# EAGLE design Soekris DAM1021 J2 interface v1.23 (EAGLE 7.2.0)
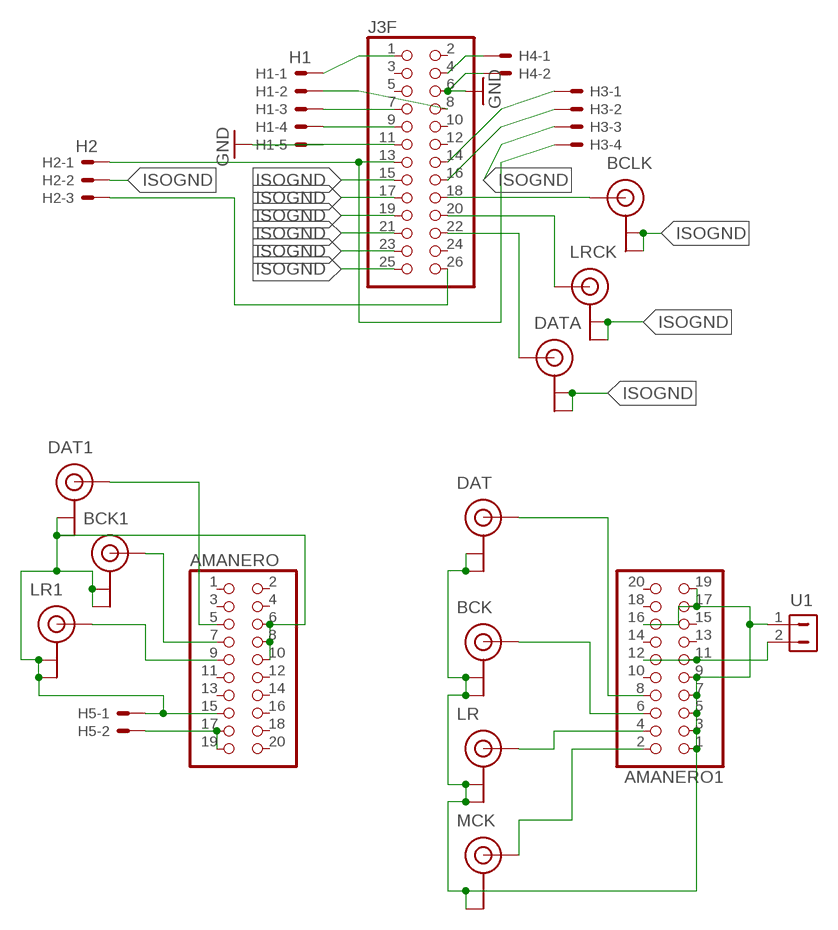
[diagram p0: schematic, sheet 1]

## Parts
AMANERO  PINHD-2X10_2.54  [2X10]
AMANERO1  PINHD-2X10_2.54  [2X10]
BCK  U.FL  [U.FL]
BCK1  U.FL  [U.FL]
BCLK  U.FL  [U.FL]
DAT  U.FL  [U.FL]
DAT1  U.FL  [U.FL]
DATA  U.FL  [U.FL]
H1  H1  22-23-2051  [22-23-2051]
H2  H2  22-23-2031  [22-23-2031]
H3  22-23-2041  [22-23-2041]
H4  22-23-2021  [22-23-2021]
H5  22-23-2021  [22-23-2021]
J3F  PINHD-2X13_2.54  [2X13]
LR  U.FL  [U.FL]
LR1  U.FL  [U.FL]
LRCK  U.FL  [U.FL]
MCK  U.FL  [U.FL]
U1  CON-2  [CON-2]

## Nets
GND: H1.5 H4.2 J3F.6 J3F.11
GNDA: AMANERO.6 AMANERO.8 AMANERO.10 AMANERO.15 BCK1.P$1(GND) BCK1.P$2(GND) DAT1.P$1(GND) DAT1.P$2(GND) H5.1 LR1.P$1(GND) LR1.P$2(GND)
H2: H2.3 J3F.26
ISOGND: BCLK.P$1(GND) BCLK.P$2(GND) DATA.P$1(GND) DATA.P$2(GND) H2.2 H3.3 J3F.15 J3F.17 J3F.19 J3F.21 J3F.23 J3F.25 LRCK.P$1(GND) LRCK.P$2(GND)
N$1: H2.1 H3.4 J3F.13
N$2: AMANERO1.2 MCK.P$3(SIGNAL)
N$3: H3.1 J3F.14
N$4: H3.2 J3F.16
N$5: BCLK.P$3(SIGNAL) J3F.18
N$6: H1.1 J3F.1
N$7: DATA.P$3(SIGNAL) J3F.22
N$8: AMANERO1.4 LR.P$3(SIGNAL)
N$9: J3F.20 LRCK.P$3(SIGNAL)
N$10: AMANERO1.8 DAT.P$3(SIGNAL)
N$11: H1.3 J3F.7
N$12: H1.2 J3F.8
N$13: H1.4 J3F.9
N$14: H4.1 J3F.4
N$15: AMANERO.17 AMANERO.19 H5.2
N$16: AMANERO1.6 BCK.P$3(SIGNAL)
N$17: AMANERO1.1 AMANERO1.3 AMANERO1.5 AMANERO1.7 AMANERO1.9 AMANERO1.16 AMANERO1.17 AMANERO1.19 BCK.P$1(GND) BCK.P$2(GND) DAT.P$1(GND) DAT.P$2(GND) LR.P$1(GND) LR.P$2(GND) MCK.P$1(GND) MCK.P$2(GND) U1.1
N$19: AMANERO.5 DAT1.P$3(SIGNAL)
N$20: AMANERO.7 BCK1.P$3(SIGNAL)
N$21: AMANERO.9 LR1.P$3(SIGNAL)
N$24: AMANERO1.11 AMANERO1.12 U1.2
Unconnected: AMANERO1.10 AMANERO1.13 AMANERO1.14 AMANERO1.15 AMANERO1.18 AMANERO1.20 AMANERO.1 AMANERO.2 AMANERO.3 AMANERO.4 AMANERO.11 AMANERO.12 AMANERO.13 AMANERO.14 AMANERO.16 AMANERO.18 AMANERO.20 J3F.2 J3F.3 J3F.5 J3F.10 J3F.12 J3F.24

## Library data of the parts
AMANERO AMANERO1 = pinhead-1:PINHD-2X10: PIN HEADER
BCK BCK1 BCLK DAT DAT1 DATA LR LR1 LRCK MCK = Dimdim:U.FL
H1 = con-molex:22-23-2051: .100" (2.54mm) Center Header - 5 Pin; MF: MOLEX; MPN: 22-23-2051; OC_FARNELL: 1462952; OC_NEWARK: 38C9178
H2 = con-molex:22-23-2031: .100" (2.54mm) Center Header - 3 Pin; MF: MOLEX; MPN: 22-23-2031; OC_FARNELL: 1462950; OC_NEWARK: 30C0862
H3 = con-molex:22-23-2041: .100" (2.54mm) Center Header - 4 Pin; MF: MOLEX; MPN: 22-23-2041; OC_FARNELL: 1462920; OC_NEWARK: 38C0355
H4 H5 = con-molex:22-23-2021: .100" (2.54mm) Center Header - 2 Pin; MF: MOLEX; MPN: 22-23-2021; OC_FARNELL: 1462926; OC_NEWARK: 25C3832
J3F = pinhead-1:PINHD-2X13: PIN HEADER
U1 = Dimdim:CON-2

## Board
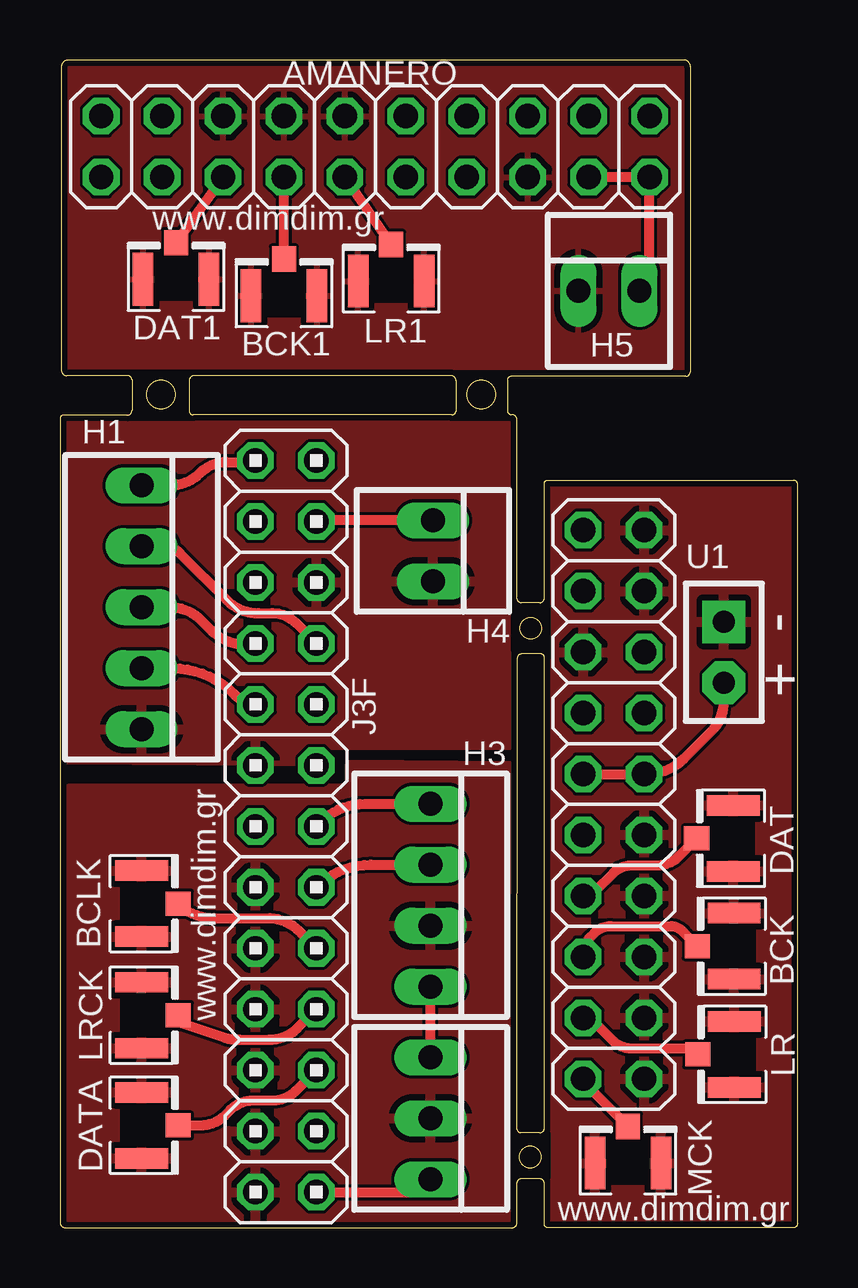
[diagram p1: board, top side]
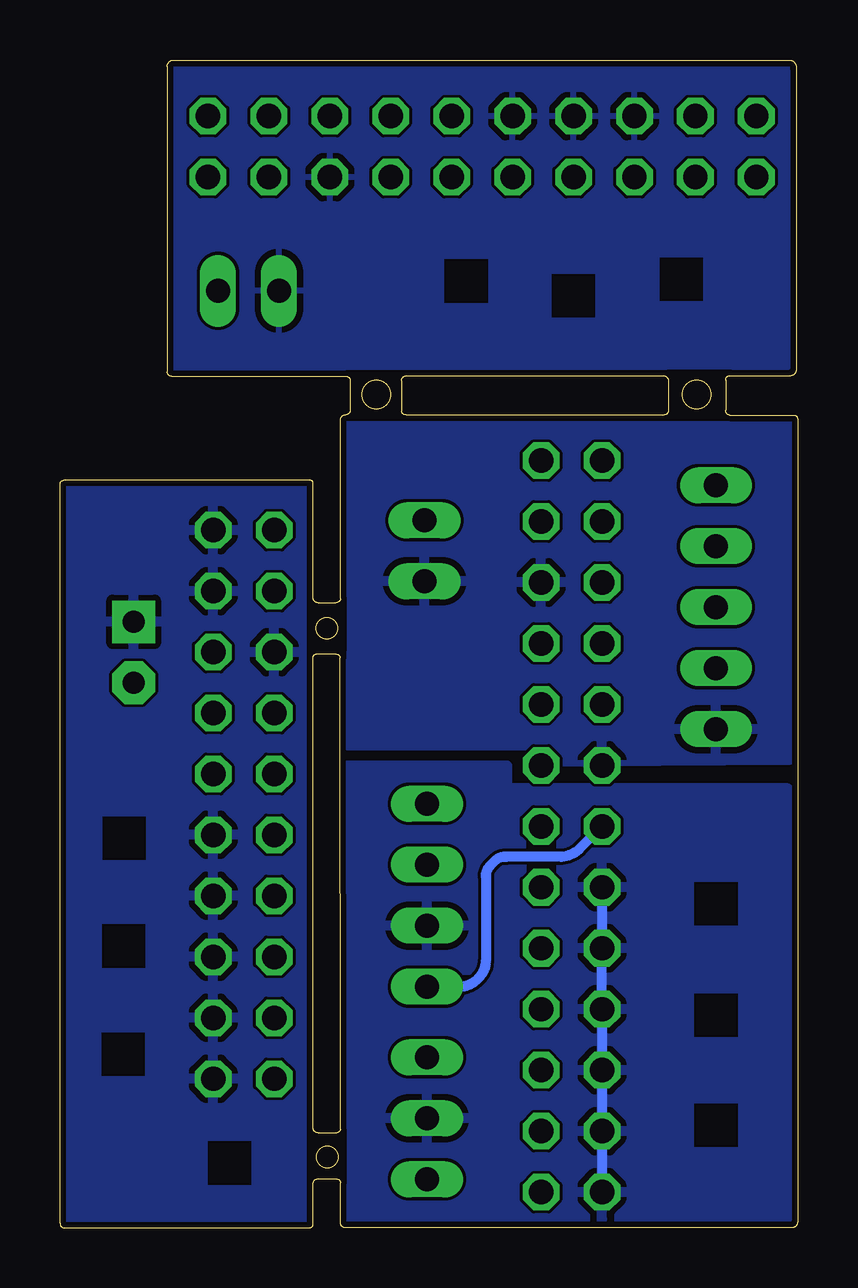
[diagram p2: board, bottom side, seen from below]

Size 30.75 x 48.66 mm. Coordinates in mm from the lower left corner, seen from the top.
Outline: 63 segments
Outline: circle at 19.6,2.95 radius 0.45
Outline: circle at 19.62,24.98 radius 0.45
Outline: circle at 4.21,34.73 radius 0.6
Outline: circle at 17.57,34.72 radius 0.6
Copper layers (1*16): Top 0.035mm / dielectric 1.5mm / Bottom 0.035mm
Design rules "dirt_cheap_dirty_boards.v1": minimum track width 5mil, minimum drill 12mil, track to track 5mil, track to pad 5mil, pad to pad 5mil, via to via 5mil, smd to smd 0mil, copper to edge 10mil, drill to drill 10mil, minimum pad ring 10mil, minimum via ring 6mil, stop-mask expansion 2mil, vias tented up to drill 25mil, thermal gap 10mil
tRestrict: area 18.8,24 to 20.4,25.9; area 18.8,2.1 to 20.4,4; area 2.9,33.6 to 5.4,35.8; area 16.3,33.6 to 18.8,35.7
bRestrict: area 18.8,2.1 to 20.4,4; area 18.8,24 to 20.4,25.9; area 2.9,33.6 to 5.4,35.8; area 16.3,33.6 to 18.8,35.7

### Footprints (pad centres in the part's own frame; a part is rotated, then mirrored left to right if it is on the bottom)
2X10 = drill 1.016 octagon: 1 -11.43,-1.27; 2 -11.43,1.27; 3 -8.89,-1.27; 4 -8.89,1.27; 5 -6.35,-1.27; 6 -6.35,1.27; 7 -3.81,-1.27; 8 -3.81,1.27; 9 -1.27,-1.27; 10 -1.27,1.27; 11 1.27,-1.27; 12 1.27,1.27; 13 3.81,-1.27; 14 3.81,1.27; 15 6.35,-1.27; 16 6.35,1.27; 17 8.89,-1.27; 18 8.89,1.27; 19 11.43,-1.27; 20 11.43,1.27
U.FL = smd 2.2 x 0.85: P$1 0,1.375; P$2 0,-1.375 | smd 1.05 x 1: P$3 1.525,0
22-23-2051 = drill 1 long: 1 -5.08,0; 2 -2.54,0; 3 0,0; 4 2.54,0; 5 5.08,0
22-23-2031 = drill 1 long: 1 -2.54,0; 2 0,0; 3 2.54,0
22-23-2041 = drill 1 long: 1 -3.81,0; 2 -1.27,0; 3 1.27,0; 4 3.81,0
22-23-2021 = drill 1 long: 1 -1.27,0; 2 1.27,0
2X13 = drill 1.016 octagon: 1 -15.24,-1.27; 2 -15.24,1.27; 3 -12.7,-1.27; 4 -12.7,1.27; 5 -10.16,-1.27; 6 -10.16,1.27; 7 -7.62,-1.27; 8 -7.62,1.27; 9 -5.08,-1.27; 10 -5.08,1.27; 11 -2.54,-1.27; 12 -2.54,1.27; 13 0,-1.27; 14 0,1.27; 15 2.54,-1.27; 16 2.54,1.27; 17 5.08,-1.27; 18 5.08,1.27; 19 7.62,-1.27; 20 7.62,1.27; 21 10.16,-1.27; 22 10.16,1.27; 23 12.7,-1.27; 24 12.7,1.27; 25 15.24,-1.27; 26 15.24,1.27
CON-2 = drill 0.914 pad 1.778 square: 1 -1.27,0 | drill 0.914 pad 1.778 octagon: 2 1.27,0

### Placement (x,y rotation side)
AMANERO  13.15,45.05 0 top
AMANERO1  23.09,17.64 90 top
BCK  28.1,11.74 180 top
BCK1  9.34,38.84 90 top
BCLK  3.4,13.51 0 top
DAT  28.07,16.23 180 top
DAT1  4.84,39.52 90 top
DATA  3.4,4.27 0 top
H1  3.4,25.86 270 top
H2  15.45,4.56 270 top
H3  15.45,13.86 270 top
H4  15.55,28.21 270 top
H5  22.89,39.04 0 top
J3F  9.42,16.73 270 top
LR  28.12,7.23 180 top
LR1  13.81,39.45 90 top
LRCK  3.4,8.86 0 top
MCK  23.68,2.7 90 top
U1  27.68,23.98 270 top

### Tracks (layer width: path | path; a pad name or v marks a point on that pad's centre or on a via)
GND
  pour Top: 0.3,33.61 18.8,33.61 18.8,20.11 11.1,20.11 11.1,19.41 0.3,19.51
  pour Bottom: 0.3,33.61 18.8,33.61 18.8,20.11 11.1,20.11 11.1,19.41 0.3,19.51
GNDA
  pour Top: 0.25,48.54 26.13,48.55 26.15,35.7 0.19,35.76
  pour Bottom: 0.25,48.54 26.13,48.55 26.15,35.7 0.19,35.76
H2
  Top 0.406: J3F.26 15.16,1.49 arc59 H2.3
ISOGND
  Bottom 0.406: J3F.15 J3F.17 J3F.19 J3F.21 J3F.23 J3F.25
  pour Top: 18.85,19.26 18.85,0.21 0.2,0.21 0.3,8.76 0.3,8.86 0.4,18.31 12.1,18.31 12.1,19.31
  pour Bottom: 0.25,0.21 0.3,4.91 0.3,8.76 0.4,18.31 12.1,18.31 12.1,19.26 18.85,19.26 18.85,0.21
N$1
  Top 0.406: H2.1 H3.4
  Bottom 0.406: J3F.13 9.03,15.85 arc45 9.85,15.46 12.14,15.46 arc-45 12.59,15.32 12.8,15.11 arc-45 13,14.63 13,11.12 arc45 13.29,10.42 13.37,10.34 arc45 14.07,10.05 H3.4
N$2
  Top 0.406: AMANERO1.2 21.82,6.08 MCK.P$3
N$3
  Top 0.406: J3F.14 10.86,16.89 arc-45 12.73,17.67 H3.1
N$4
  Top 0.406: J3F.16 arc-45 12.96,15.13 H3.2
N$5
  Top 0.406: BCLK.P$3 arc46 6.41,12.91 8.74,12.91 arc-45 10.09,12.25 J3F.18
N$6
  Top 0.254: 8.09,31.91 J3F.1
  Top 0.406: H1.1 4.6,30.94 arc45 5.84,31.45 arc-45 6.95,31.91 8.09,31.91
N$7
  Top 0.406: DATA.P$3 5.87,4.27 arc45 6.88,4.69 7.11,4.92 arc-45 8.05,5.31 8.88,5.31 arc45 9.82,5.7 J3F.22
N$8
  Top 0.406: AMANERO1.4 arc-45 22.3,8.55 23.03,7.82 arc45 23.78,7.48 26.32,7.48 LR.P$3
N$9
  Top 0.254: LRCK.P$3 4.95,8.56
  Top 0.406: 4.95,8.56 6.88,7.92 arc18 7.47,7.84 8.72,7.84 arc45 9.89,8.31 J3F.20
N$10
  Top 0.406: AMANERO1.8 arc45 22.33,14.04 23.09,14.8 arc-45 23.79,15.1 24.85,15.1 arc45 25.8,15.48 DAT.P$3
N$11
  Top 0.254: 8.11,24.31 J3F.7
  Top 0.406: H1.3 4.58,25.86 arc-45 5.9,25.31 6.32,24.89 arc45 7.71,24.31 8.11,24.31
N$12
  Top 0.406: H1.2 4.31,28.4 arc-45 5,28.11 6.96,26.15 arc45 8.26,25.61 8.86,25.61 arc-45 9.84,25.2 J3F.8
N$13
  Top 0.254: H1.4
  Top 0.406: H1.4 4.69,23.31 arc-45 7.27,22.24 7.38,22.13 arc45 J3F.9
N$14
  Top 0.254: 10.74,29.48 J3F.4
  Top 0.406: H4.1 10.74,29.48
N$15
  Top 0.406: AMANERO.17 AMANERO.19 24.58,39.04 H5.2
N$16
  Top 0.406: AMANERO1.6 21.82,11.35 arc-45 22.11,12.12 22.3,12.3 arc-45 22.97,12.57 25.49,12.57 arc-45 25.99,12.32 BCK.P$3
N$17
  pour Top: 20.4,30.94 30.57,30.94 30.55,0.21 20.4,0.21
  pour Bottom: 20.4,0.21 30.55,0.21 30.57,30.94 20.4,30.94
N$19
  Top 0.406: DAT1.P$3 AMANERO.5
N$20
  Top 0.406: BCK1.P$3 AMANERO.7
N$21
  Top 0.406: LR1.P$3 AMANERO.9
N$24
  Top 0.406: AMANERO1.12 AMANERO1.11 24.45,18.91 arc45 26.04,19.57 27.18,20.71 arc45 27.68,21.92 U1.2

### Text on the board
tNames: www.dimdim.gr | - | + | www.dimdim.gr | www.dimdim.gr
